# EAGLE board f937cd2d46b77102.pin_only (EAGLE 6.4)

Size 154.94 x 25.4 mm. Coordinates in mm from the lower left corner, seen from the top.
Outline: 0,0 0,25.4 154.94,25.4 154.94,0 0,0
Copper layers (1*16): Top 0.035mm / dielectric 1.5mm / Bottom 0.035mm
Design rules "adafruit_rules_1": minimum track width 8mil, minimum drill 15.5mil, track to track 8mil, track to pad 8mil, pad to pad 8mil, via to via 8mil, smd to smd 8mil, copper to edge 10mil, drill to drill 8mil, minimum pad ring 10mil, minimum via ring 8mil, stop-mask expansion 4mil, vias tented up to drill 25mil, thermal gap 10mil

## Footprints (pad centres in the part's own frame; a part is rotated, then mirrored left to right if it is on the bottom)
0201 = smd 0.3 x 0.3: P$1 -0.3,0; P$2 0.3,0
0402 = smd 0.5 x 0.6: 1 -0.5,0; 2 0.5,0
0603 = smd 0.6 x 0.9: 1 -0.75,0; 2 0.75,0
0805 = smd 1.2 x 1.3: 1 -1.05,0; 2 1.05,0
1206 = smd 0.9 x 1.6: 1 -1.45,0; 2 1.45,0
1210 = smd 1 x 2.8: 1 -1.5,0; 2 1.5,0
2010 = smd 1 x 2.8: P$1 -2.3,0; P$2 2.3,0
DPAK = smd 1.6 x 3: 1 -2.28,-5.31; 3 2.28,-5.31 | smd 4.826 x 5.715: 4 0,1.588
D2PAK = smd 1.6 x 3.5: 1 -2.54,-8.275; 3 2.54,-8.275 | smd 12.2 x 9.75: TAB 0,2
SOT223 = smd 1.219 x 2.235: 1 -2.311,-3.099; 2 0,-3.099; 3 2.311,-3.099 | smd 3.6 x 2.2: 4 0,3.099
SOT89 = smd 0.58 x 1.2: 1 -1.5,-1.8; 2 0,-1.8; 3 1.5,-1.8 | smd 2 x 2: 4 0,1.3
SOT23-5 = smd 0.55 x 1.2: 1 -0.95,-1.3; 2 0,-1.3; 3 0.95,-1.3; 4 0.95,1.3; 5 -0.95,1.3
SOT23-3 = smd 0.8 x 0.9: 1 -0.95,-1; 2 0.95,-1; 3 0,1.1
SC70 = smd 0.4 x 0.75: 1 -0.65,-0.825; 2 0,-0.825; 3 0.65,-0.825; 4 0.65,0.825; 5 -0.65,0.825
CRYSTAL-SMD-5X3.2 = smd 1.8 x 1.2: 1 -2,-1.2; 2 2,-1.2; 3 2,1.2; 4 -2,1.2
CRYSTAL-SMD-3.2X2.5 = smd 1.4 x 1.2: 1 -1.2,-0.95; 2 1.2,-0.95; 3 1.2,0.95; 4 -1.2,0.95
CRYSTAL-SMD-2.5X2 = smd 1.05 x 0.9: 1 -0.795,-0.6; 2 0.795,-0.6; 3 0.795,0.6; 4 -0.795,0.6
HC49UP = smd 5.334 x 1.93: 1 -4.826,0; 2 4.826,0
XTAL-2X1.2 = smd 1 x 1.4: P$1 -0.85,0; P$2 0.85,0
MICROMELF-R = smd 0.8 x 1.2: A 0.8,0; C -0.8,0
SC79_INFINEON = smd 0.35 x 0.35: A 0.675,0; C -0.675,0
SMA-DIODE = smd 1.27 x 1.47: A -2.15,0; C 2.15,0
SMB-DIODE = smd 2.4 x 2.4: A 2.2,0; C -2.2,0
SMC = smd 2.8 x 3.8: A 3.7,0; C -3.7,0
ALL-HOLES = hole 3.26: 43.004,-1.63 | hole 2.91: 39.118,-1.455 | hole 2.59: 35.569,-1.295 | hole 2.3: 32.324,-1.15 | hole 2.05: 29.349,-1.025 | hole 1.83: 26.608,-0.915 | hole 1.63: 24.078,-0.815 | hole 1.45: 21.738,-0.725 | hole 1.29: 19.569,-0.645 | hole 1.15: 17.549,-0.575 | hole 1.02: 15.664,-0.51 | hole 0.912: 13.898,-0.456 | hole 0.812: 12.236,-0.406 | hole 0.723: 10.668,-0.361 | hole 0.644: 9.144,-0.322 | hole 0.573: 7.62,-0.286 | hole 0.511: 6.096,-0.256 | hole 0.455: 4.572,-0.228 | hole 0.405: 3.048,-0.203 | hole 0.361: 1.524,-0.18 | hole 0.321: 0,-0.161
SOD-128 = smd 1.4 x 2.1: A 2.2,0; C -2.2,0
SOD-323 = smd 0.63 x 0.83: 1 -1.15,0; 2 1.15,0
SOD80C = smd 1.4 x 1.8: A 1.7,0; C -1.7,0
QFN-24 = smd 0.8 x 0.25: 1 -2,1.25; 2 -2,0.75; 3 -2,0.25; 4 -2,-0.25; 5 -2,-0.75; 6 -2,-1.25; 13 2,-1.25; 14 2,-0.75; 15 2,-0.25; 16 2,0.25; 17 2,0.75; 18 2,1.25 | smd 0.25 x 0.8: 7 -1.25,-2; 8 -0.75,-2; 9 -0.25,-2; 10 0.25,-2; 11 0.75,-2; 12 1.25,-2; 19 1.25,2; 20 0.75,2; 21 0.25,2; 22 -0.25,2; 23 -0.75,2; 24 -1.25,2
TSSOP16 = smd 0.35 x 1.6: 1 -2.225,-2.85; 2 -1.575,-2.85; 3 -0.925,-2.85; 4 -0.275,-2.85; 5 0.375,-2.85; 6 1.025,-2.85; 7 1.675,-2.85; 8 2.325,-2.85; 9 2.325,3.05; 10 1.675,3.05; 11 1.025,3.05; 12 0.375,3.05; 13 -0.275,3.05; 14 -0.925,3.05; 15 -1.575,3.05; 16 -2.225,3.05
SO08 = smd 0.61 x 2.21: 1 -1.905,-2.616; 2 -0.635,-2.616; 3 0.635,-2.616; 4 1.905,-2.616; 5 1.905,2.616; 6 0.635,2.616; 7 -0.635,2.616; 8 -1.905,2.616
TQFP32-5MM = smd 1.143 x 0.254: 1 -3.5,1.75; 2 -3.5,1.25; 3 -3.5,0.75; 4 -3.5,0.25; 5 -3.5,-0.25; 6 -3.5,-0.75; 7 -3.5,-1.25; 8 -3.5,-1.75; 17 3.5,-1.75; 18 3.5,-1.25; 19 3.5,-0.75; 20 3.5,-0.25; 21 3.5,0.25; 22 3.5,0.75; 23 3.5,1.25; 24 3.5,1.75 | smd 0.254 x 1.143: 9 -1.75,-3.5; 10 -1.25,-3.5; 11 -0.75,-3.5; 12 -0.25,-3.5; 13 0.25,-3.5; 14 0.75,-3.5; 15 1.25,-3.5; 16 1.75,-3.5; 25 1.75,3.5; 26 1.25,3.5; 27 0.75,3.5; 28 0.25,3.5; 29 -0.25,3.5; 30 -0.75,3.5; 31 -1.25,3.5; 32 -1.75,3.5
TQFP100 = smd 1.5 x 0.3: 1 -8,6; 2 -8,5.5; 3 -8,5; 4 -8,4.5; 5 -8,4; 6 -8,3.5; 7 -8,3; 8 -8,2.5; 9 -8,2; 10 -8,1.5; 11 -8,1; 12 -8,0.5; 13 -8,0; 14 -8,-0.5; 15 -8,-1; 16 -8,-1.5; 17 -8,-2; 18 -8,-2.5; 19 -8,-3; 20 -8,-3.5; 21 -8,-4; 22 -8,-4.5; 23 -8,-5; 24 -8,-5.5; 25 -8,-6; 51 8,-6; 52 8,-5.5; 53 8,-5; 54 8,-4.5; 55 8,-4; 56 8,-3.5; 57 8,-3; 58 8,-2.5; 59 8,-2; 60 8,-1.5; 61 8,-1; 62 8,-0.5; 63 8,0; 64 8,0.5; 65 8,1; 66 8,1.5; 67 8,2; 68 8,2.5; 69 8,3; 70 8,3.5; 71 8,4; 72 8,4.5; 73 8,5; 74 8,5.5; 75 8,6 | smd 0.3 x 1.5: 26 -6,-8; 27 -5.5,-8; 28 -5,-8; 29 -4.5,-8; 30 -4,-8; 31 -3.5,-8; 32 -3,-8; 33 -2.5,-8; 34 -2,-8; 35 -1.5,-8; 36 -1,-8; 37 -0.5,-8; 38 0,-8; 39 0.5,-8; 40 1,-8; 41 1.5,-8; 42 2,-8; 43 2.5,-8; 44 3,-8; 45 3.5,-8; 46 4,-8; 47 4.5,-8; 48 5,-8; 49 5.5,-8; 50 6,-8; 76 6,8; 77 5.5,8; 78 5,8; 79 4.5,8; 80 4,8; 81 3.5,8; 82 3,8; 83 2.5,8; 84 2,8; 85 1.5,8; 86 1,8; 87 0.5,8; 88 0,8; 89 -0.5,8; 90 -1,8; 91 -1.5,8; 92 -2,8; 93 -2.5,8; 94 -3,8; 95 -3.5,8; 96 -4,8; 97 -4.5,8; 98 -5,8; 99 -5.5,8; 100 -6,8
TSOP-66 = smd 0.35 x 0.8: P$1 -10.4,-5.7; P$2 -9.75,-5.7; P$3 -9.1,-5.7; P$4 -8.45,-5.7; P$5 -7.8,-5.7; P$6 -7.15,-5.7; P$7 -6.5,-5.7; P$8 -5.85,-5.7; P$9 -5.2,-5.7; P$10 -4.55,-5.7; P$11 -3.9,-5.7; P$12 -3.25,-5.7; P$13 -2.6,-5.7; P$14 -1.95,-5.7; P$15 -1.3,-5.7; P$16 -0.65,-5.7; P$17 0,-5.7; P$18 0.65,-5.7; P$19 1.3,-5.7; P$20 1.95,-5.7; P$21 2.6,-5.7; P$22 3.25,-5.7; P$23 3.9,-5.7; P$24 4.55,-5.7; P$25 5.2,-5.7; P$26 5.85,-5.7; P$27 6.5,-5.7; P$28 7.15,-5.7; P$29 7.8,-5.7; P$30 8.45,-5.7; P$31 9.1,-5.7; P$32 9.75,-5.7; P$33 10.4,-5.7; P$34 10.4,5.7; P$35 9.75,5.7; P$36 9.1,5.7; P$37 8.45,5.7; P$38 7.8,5.7; P$39 7.15,5.7; P$40 6.5,5.7; P$41 5.85,5.7; P$42 5.2,5.7; P$43 4.55,5.7; P$44 3.9,5.7; P$45 3.25,5.7; P$46 2.6,5.7; P$47 1.95,5.7; P$48 1.3,5.7; P$49 0.65,5.7; P$50 0,5.7; P$51 -0.65,5.7; P$52 -1.3,5.7; P$53 -1.95,5.7; P$54 -2.6,5.7; P$55 -3.25,5.7; P$56 -3.9,5.7; P$57 -4.55,5.7; P$58 -5.2,5.7; P$59 -5.85,5.7; P$60 -6.5,5.7; P$61 -7.15,5.7; P$62 -7.8,5.7; P$63 -8.45,5.7; P$64 -9.1,5.7; P$65 -9.75,5.7; P$66 -10.4,5.7
BGA-0.8MM-P-19X19 = smd 0.35 x 0.35: P$1 -4.4,-4.4; P$2 -4.4,-3.6; P$3 -3.6,-3.6; P$4 -3.6,-4.4; P$5 -2.8,-4.4; P$6 -2.8,-3.6; P$7 -4.4,-2.8; P$8 -3.6,-2.8; P$9 -2.8,-2.8; P$10 -4.4,-2; P$11 -3.6,-2; P$12 -2.8,-2; P$13 -2,-2; P$14 -2,-2.8; P$15 -2,-3.6; P$16 -2,-4.4; P$17 -4.4,-1.2; P$18 -3.6,-1.2; P$19 -2.8,-1.2; P$20 -2,-1.2; P$21 -1.2,-1.2; P$22 -1.2,-2; P$23 -1.2,-2.8; P$24 -1.2,-3.6; P$25 -1.2,-4.4; P$26 -3.6,-7.6; P$27 -2.8,-7.6; P$28 -3.6,-6.8; P$29 -2.8,-6.8; P$30 -3.6,-6; P$31 -2.8,-6; P$32 -2,-6; P$33 -2,-6.8; P$34 -2,-7.6; P$35 -3.6,-5.2; P$36 -2.8,-5.2; P$37 -2,-5.2; P$38 -1.2,-5.2; P$39 -1.2,-6; P$40 -1.2,-6.8; P$41 -1.2,-7.6; P$42 -7.6,-3.6; P$43 -6.8,-3.6; P$44 -7.6,-2.8; P$45 -6.8,-2.8; P$46 -7.6,-2; P$47 -6.8,-2; P$48 -6,-2; P$49 -6,-2.8; P$50 -6,-3.6; P$51 -7.6,-1.2; P$52 -6.8,-1.2; P$53 -6,-1.2; P$54 -5.2,-1.2; P$55 -5.2,-2; P$56 -5.2,-2.8; P$57 -5.2,-3.6; P$58 -7.6,-7.6; P$59 -6.8,-7.6; P$60 -7.6,-6.8; P$61 -6.8,-6.8; P$62 -7.6,-6; P$63 -6.8,-6; P$64 -6,-6; P$65 -6,-6.8; P$66 -6,-7.6; P$67 -7.6,-5.2; P$68 -6.8,-5.2; P$69 -6,-5.2; P$70 -5.2,-5.2; P$71 -5.2,-6; P$72 -5.2,-6.8; P$73 -5.2,-7.6; P$74 -7.6,-4.4; P$75 -6.8,-4.4; P$76 -6,-4.4; P$77 -5.2,-4.4; P$78 -4.4,-5.2; P$79 -4.4,-6; P$80 -4.4,-6.8; P$81 -4.4,-7.6; P$82 2.8,-4.4; P$83 2.8,-3.6; P$84 3.6,-3.6; P$85 3.6,-4.4; P$86 4.4,-4.4; P$87 4.4,-3.6; P$88 2.8,-2.8; P$89 3.6,-2.8; P$90 4.4,-2.8; P$91 2.8,-2; P$92 3.6,-2; P$93 4.4,-2; P$94 5.2,-2; P$95 5.2,-2.8; P$96 5.2,-3.6; P$97 5.2,-4.4; P$98 2.8,-1.2; P$99 3.6,-1.2; P$100 4.4,-1.2; P$101 5.2,-1.2; P$102 6,-1.2; P$103 6,-2; P$104 6,-2.8; P$105 6,-3.6; P$106 6,-4.4; P$107 3.6,-7.6; P$108 4.4,-7.6; P$109 3.6,-6.8; P$110 4.4,-6.8; P$111 3.6,-6; P$112 4.4,-6; P$113 5.2,-6; P$114 5.2,-6.8; P$115 5.2,-7.6; P$116 3.6,-5.2; P$117 4.4,-5.2; P$118 5.2,-5.2; P$119 6,-5.2; P$120 6,-6; P$121 6,-6.8; P$122 6,-7.6; P$123 -0.4,-3.6; P$124 0.4,-3.6; P$125 -0.4,-2.8; P$126 0.4,-2.8; P$127 -0.4,-2; P$128 0.4,-2; P$129 1.2,-2; P$130 1.2,-2.8; P$131 1.2,-3.6; P$132 -0.4,-1.2; P$133 0.4,-1.2; P$134 1.2,-1.2; P$135 2,-1.2; P$136 2,-2; P$137 2,-2.8; P$138 2,-3.6; P$139 -0.4,-7.6; P$140 0.4,-7.6; P$141 -0.4,-6.8; P$142 0.4,-6.8; P$143 -0.4,-6; P$144 0.4,-6; P$145 1.2,-6; P$146 1.2,-6.8; P$147 1.2,-7.6; P$148 -0.4,-5.2; P$149 0.4,-5.2; P$150 1.2,-5.2; P$151 2,-5.2; P$152 2,-6; P$153 2,-6.8; P$154 2,-7.6; P$155 -0.4,-4.4; P$156 0.4,-4.4; P$157 1.2,-4.4; P$158 2,-4.4; P$159 2.8,-5.2; P$160 2.8,-6; P$161 2.8,-6.8; P$162 2.8,-7.6; P$163 -4.4,2.8; P$164 -4.4,3.6; P$165 -3.6,3.6; P$166 -3.6,2.8; P$167 -2.8,2.8; P$168 -2.8,3.6; P$169 -4.4,4.4; P$170 -3.6,4.4; P$171 -2.8,4.4; P$172 -4.4,5.2; P$173 -3.6,5.2; P$174 -2.8,5.2; P$175 -2,5.2; P$176 -2,4.4; P$177 -2,3.6; P$178 -2,2.8; P$179 -4.4,6; P$180 -3.6,6; P$181 -2.8,6; P$182 -2,6; P$183 -1.2,6; P$184 -1.2,5.2; P$185 -1.2,4.4; P$186 -1.2,3.6; P$187 -1.2,2.8; P$188 -3.6,-0.4; P$189 -2.8,-0.4; P$190 -3.6,0.4; P$191 -2.8,0.4; P$192 -3.6,1.2; P$193 -2.8,1.2; P$194 -2,1.2; P$195 -2,0.4; P$196 -2,-0.4; P$197 -3.6,2; P$198 -2.8,2; P$199 -2,2; P$200 -1.2,2; P$201 -1.2,1.2; P$202 -1.2,0.4; P$203 -1.2,-0.4; P$204 -7.6,3.6; P$205 -6.8,3.6; P$206 -7.6,4.4; P$207 -6.8,4.4; P$208 -7.6,5.2; P$209 -6.8,5.2; P$210 -6,5.2; P$211 -6,4.4; P$212 -6,3.6; P$213 -7.6,6; P$214 -6.8,6; P$215 -6,6; P$216 -5.2,6; P$217 -5.2,5.2; P$218 -5.2,4.4; P$219 -5.2,3.6; P$220 -7.6,-0.4; P$221 -6.8,-0.4; P$222 -7.6,0.4; P$223 -6.8,0.4; P$224 -7.6,1.2; P$225 -6.8,1.2; P$226 -6,1.2; P$227 -6,0.4; P$228 -6,-0.4; P$229 -7.6,2; P$230 -6.8,2; P$231 -6,2; P$232 -5.2,2; P$233 -5.2,1.2; P$234 -5.2,0.4; P$235 -5.2,-0.4; P$236 -7.6,2.8; P$237 -6.8,2.8; P$238 -6,2.8; P$239 -5.2,2.8; P$240 -4.4,2; P$241 -4.4,1.2; P$242 -4.4,0.4; P$243 -4.4,-0.4; P$244 2.8,2.8; P$245 2.8,3.6; P$246 3.6,3.6; P$247 3.6,2.8; P$248 4.4,2.8; P$249 4.4,3.6; P$250 2.8,4.4; P$251 3.6,4.4; P$252 4.4,4.4; P$253 2.8,5.2; P$254 3.6,5.2; P$255 4.4,5.2; P$256 5.2,5.2; P$257 5.2,4.4; P$258 5.2,3.6; P$259 5.2,2.8; P$260 2.8,6; P$261 3.6,6; P$262 4.4,6; P$263 5.2,6; P$264 6,6; P$265 6,5.2; P$266 6,4.4; P$267 6,3.6; P$268 6,2.8; P$269 3.6,-0.4; P$270 4.4,-0.4; P$271 3.6,0.4; P$272 4.4,0.4; P$273 3.6,1.2; P$274 4.4,1.2; P$275 5.2,1.2; P$276 5.2,0.4; P$277 5.2,-0.4; P$278 3.6,2; P$279 4.4,2; P$280 5.2,2; P$281 6,2; P$282 6,1.2; P$283 6,0.4; P$284 6,-0.4; P$285 -0.4,3.6; P$286 0.4,3.6; P$287 -0.4,4.4; P$288 0.4,4.4; P$289 -0.4,5.2; P$290 0.4,5.2; P$291 1.2,5.2; P$292 1.2,4.4; P$293 1.2,3.6; P$294 -0.4,6; P$295 0.4,6; P$296 1.2,6; P$297 2,6; P$298 2,5.2; P$299 2,4.4; P$300 2,3.6; P$301 -0.4,-0.4; P$302 0.4,-0.4; P$303 -0.4,0.4; P$304 0.4,0.4; P$305 -0.4,1.2; P$306 0.4,1.2; P$307 1.2,1.2; P$308 1.2,0.4; P$309 1.2,-0.4; P$310 -0.4,2; P$311 0.4,2; P$312 1.2,2; P$313 2,2; P$314 2,1.2; P$315 2,0.4; P$316 2,-0.4; P$317 -0.4,2.8; P$318 0.4,2.8; P$319 1.2,2.8; P$320 2,2.8; P$321 2.8,2; P$322 2.8,1.2; P$323 2.8,0.4; P$324 2.8,-0.4; P$325 -4.4,6.8; P$326 -3.6,6.8; P$327 -2.8,6.8; P$328 -4.4,7.6; P$329 -3.6,7.6; P$330 -2.8,7.6; P$331 -2,7.6; P$332 -2,6.8; P$338 -1.2,7.6; P$339 -1.2,6.8; P$340 -7.6,6.8; P$341 -6.8,6.8; P$342 -7.6,7.6; P$343 -6.8,7.6; P$344 -6,7.6; P$345 -6,6.8; P$350 -5.2,7.6; P$351 -5.2,6.8; P$352 2.8,6.8; P$353 3.6,6.8; P$354 4.4,6.8; P$355 2.8,7.6; P$356 3.6,7.6; P$357 4.4,7.6; P$358 5.2,7.6; P$359 5.2,6.8; P$365 6,7.6; P$366 6,6.8; P$367 -0.4,6.8; P$368 0.4,6.8; P$369 -0.4,7.6; P$370 0.4,7.6; P$371 1.2,7.6; P$372 1.2,6.8; P$377 2,7.6; P$378 2,6.8; P$379 6.8,-4.4; P$380 6.8,-3.6; P$381 6.8,-2.8; P$382 6.8,-2; P$383 7.6,-2; P$384 7.6,-2.8; P$385 7.6,-3.6; P$386 7.6,-4.4; P$387 6.8,-1.2; P$388 7.6,-1.2; P$394 6.8,-7.6; P$395 6.8,-6.8; P$396 6.8,-6; P$397 7.6,-6; P$398 7.6,-6.8; P$399 7.6,-7.6; P$400 6.8,-5.2; P$401 7.6,-5.2; P$406 6.8,2.8; P$407 6.8,3.6; P$408 6.8,4.4; P$409 6.8,5.2; P$410 7.6,5.2; P$411 7.6,4.4; P$412 7.6,3.6; P$413 7.6,2.8; P$414 6.8,6; P$415 7.6,6; P$421 6.8,-0.4; P$422 6.8,0.4; P$423 6.8,1.2; P$424 7.6,1.2; P$425 7.6,0.4; P$426 7.6,-0.4; P$427 6.8,2; P$428 7.6,2; P$433 6.8,6.8; P$434 6.8,7.6; P$435 7.6,7.6; P$436 7.6,6.8
TQFP-100-12X12MM = smd 1.5 x 0.2: 1 -6.7,4.8; 2 -6.7,4.4; 3 -6.7,4; 4 -6.7,3.6; 5 -6.7,3.2; 6 -6.7,2.8; 7 -6.7,2.4; 8 -6.7,2; 9 -6.7,1.6; 10 -6.7,1.2; 11 -6.7,0.8; 12 -6.7,0.4; 13 -6.7,0; 14 -6.7,-0.4; 15 -6.7,-0.8; 16 -6.7,-1.2; 17 -6.7,-1.6; 18 -6.7,-2; 19 -6.7,-2.4; 20 -6.7,-2.8; 21 -6.7,-3.2; 22 -6.7,-3.6; 23 -6.7,-4; 24 -6.7,-4.4; 25 -6.7,-4.8; 51 6.7,-4.8; 52 6.7,-4.4; 53 6.7,-4; 54 6.7,-3.6; 55 6.7,-3.2; 56 6.7,-2.8; 57 6.7,-2.4; 58 6.7,-2; 59 6.7,-1.6; 60 6.7,-1.2; 61 6.7,-0.8; 62 6.7,-0.4; 63 6.7,0; 64 6.7,0.4; 65 6.7,0.8; 66 6.7,1.2; 67 6.7,1.6; 68 6.7,2; 69 6.7,2.4; 70 6.7,2.8; 71 6.7,3.2; 72 6.7,3.6; 73 6.7,4; 74 6.7,4.4; 75 6.7,4.8 | smd 0.2 x 1.5: 26 -4.8,-6.7; 27 -4.4,-6.7; 28 -4,-6.7; 29 -3.6,-6.7; 30 -3.2,-6.7; 31 -2.8,-6.7; 32 -2.4,-6.7; 33 -2,-6.7; 34 -1.6,-6.7; 35 -1.2,-6.7; 36 -0.8,-6.7; 37 -0.4,-6.7; 38 0,-6.7; 39 0.4,-6.7; 40 0.8,-6.7; 41 1.2,-6.7; 42 1.6,-6.7; 43 2,-6.7; 44 2.4,-6.7; 45 2.8,-6.7; 46 3.2,-6.7; 47 3.6,-6.7; 48 4,-6.7; 49 4.4,-6.7; 50 4.8,-6.7; 76 4.8,6.7; 77 4.4,6.7; 78 4,6.7; 79 3.6,6.7; 80 3.2,6.7; 81 2.8,6.7; 82 2.4,6.7; 83 2,6.7; 84 1.6,6.7; 85 1.2,6.7; 86 0.8,6.7; 87 0.4,6.7; 88 0,6.7; 89 -0.4,6.7; 90 -0.8,6.7; 91 -1.2,6.7; 92 -1.6,6.7; 93 -2,6.7; 94 -2.4,6.7; 95 -2.8,6.7; 96 -3.2,6.7; 97 -3.6,6.7; 98 -4,6.7; 99 -4.4,6.7; 100 -4.8,6.7
TQFP32-08 = smd 1.27 x 0.559: 1 -4.293,2.8; 2 -4.293,2; 3 -4.293,1.2; 4 -4.293,0.4; 5 -4.293,-0.4; 6 -4.293,-1.2; 7 -4.293,-2; 8 -4.293,-2.8; 17 4.293,-2.8; 18 4.293,-2; 19 4.293,-1.2; 20 4.293,-0.4; 21 4.293,0.4; 22 4.293,1.2; 23 4.293,2; 24 4.293,2.8 | smd 0.559 x 1.27: 9 -2.8,-4.293; 10 -2,-4.293; 11 -1.2,-4.293; 12 -0.4,-4.293; 13 0.4,-4.293; 14 1.2,-4.293; 15 2,-4.293; 16 2.8,-4.293; 25 2.8,4.293; 26 2,4.293; 27 1.2,4.293; 28 0.4,4.293; 29 -0.4,4.293; 30 -1.2,4.293; 31 -2,4.293; 32 -2.8,4.293
BGA-96-14X8MM = smd 0.45 x 0.45: P$1 1.6,6; P$2 2.4,6; P$3 3.2,6; P$4 1.6,5.2; P$5 2.4,5.2; P$6 3.2,5.2; P$7 1.6,4.4; P$8 2.4,4.4; P$9 3.2,4.4; P$10 1.6,3.6; P$11 2.4,3.6; P$12 3.2,3.6; P$13 1.6,2.8; P$14 2.4,2.8; P$15 3.2,2.8; P$16 1.6,2; P$17 2.4,2; P$18 3.2,2; P$19 1.6,1.2; P$20 2.4,1.2; P$21 3.2,1.2; P$22 1.6,0.4; P$23 2.4,0.4; P$24 3.2,0.4; P$25 1.6,-0.4; P$26 2.4,-0.4; P$27 3.2,-0.4; P$28 1.6,-1.2; P$29 2.4,-1.2; P$30 3.2,-1.2; P$31 1.6,-2; P$32 2.4,-2; P$33 3.2,-2; P$34 1.6,-2.8; P$35 2.4,-2.8; P$36 3.2,-2.8; P$37 1.6,-3.6; P$38 2.4,-3.6; P$39 3.2,-3.6; P$40 1.6,-4.4; P$41 2.4,-4.4; P$42 3.2,-4.4; P$43 1.6,-5.2; P$44 2.4,-5.2; P$45 3.2,-5.2; P$46 1.6,-6; P$47 2.4,-6; P$48 3.2,-6; P$49 -3.2,6; P$50 -2.4,6; P$51 -1.6,6; P$52 -3.2,5.2; P$53 -2.4,5.2; P$54 -1.6,5.2; P$55 -3.2,4.4; P$56 -2.4,4.4; P$57 -1.6,4.4; P$58 -3.2,3.6; P$59 -2.4,3.6; P$60 -1.6,3.6; P$61 -3.2,2.8; P$62 -2.4,2.8; P$63 -1.6,2.8; P$64 -3.2,2; P$65 -2.4,2; P$66 -1.6,2; P$67 -3.2,1.2; P$68 -2.4,1.2; P$69 -1.6,1.2; P$70 -3.2,0.4; P$71 -2.4,0.4; P$72 -1.6,0.4; P$73 -3.2,-0.4; P$74 -2.4,-0.4; P$75 -1.6,-0.4; P$76 -3.2,-1.2; P$77 -2.4,-1.2; P$78 -1.6,-1.2; P$79 -3.2,-2; P$80 -2.4,-2; P$81 -1.6,-2; P$82 -3.2,-2.8; P$83 -2.4,-2.8; P$84 -1.6,-2.8; P$85 -3.2,-3.6; P$86 -2.4,-3.6; P$87 -1.6,-3.6; P$88 -3.2,-4.4; P$89 -2.4,-4.4; P$90 -1.6,-4.4; P$91 -3.2,-5.2; P$92 -2.4,-5.2; P$93 -1.6,-5.2; P$94 -3.2,-6; P$95 -2.4,-6; P$96 -1.6,-6

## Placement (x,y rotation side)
E$1  [EDGE-MILLIMETERS]  1.2,0 0 top
E$2  [EDGE-MILLIMETERS]  11.2,0 0 top
E$3  [EDGE-MILLIMETERS]  21.2,0 0 top
E$4  [EDGE-MILLIMETERS]  31.2,0 0 top
E$5  [EDGE-MILLIMETERS]  41.2,0 0 top
E$6  [EDGE-MILLIMETERS]  51.2,0 0 top
E$7  [EDGE-MILLIMETERS]  61.2,0 0 top
E$8  [EDGE-MILLIMETERS]  71.2,0 0 top
E$9  [EDGE-MILLIMETERS]  81.2,0 0 top
E$10  [EDGE-MILLIMETERS]  91.2,0 0 top
E$11  [EDGE-MILLIMETERS]  101.2,0 0 top
E$12  [EDGE-MILLIMETERS]  111.2,0 0 top
E$13  [EDGE-MILLIMETERS]  121.2,0 0 top
E$14  [EDGE-MILLIMETERS]  131.2,0 0 top
E$15  [EDGE-MILLIMETERS]  141.2,0 0 top
E$16  [0201]  19.05,10.46 90 top
E$17  [EDGE-INCHES-EIGTH]  1.27,25.4 0 top
E$18  [EDGE-INCHES-EIGTH]  26.67,25.4 0 top
E$19  [EDGE-INCHES-EIGTH]  52.07,25.4 0 top
E$20  [EDGE-INCHES-EIGTH]  77.47,25.4 0 top
E$21  [EDGE-INCHES-EIGTH]  102.87,25.4 0 top
E$22  [EDGE-INCHES-EIGTH]  128.27,25.4 0 top
E$23  [0402]  20.57,10.16 90 top
E$24  [0603]  22.1,9.86 90 top
E$25  [0805]  23.62,9.27 90 top
E$26  [1206]  25.58,9.02 90 top
E$27  [1210]  28.3,8.92 270 top
E$28  [2010]  31.62,8.13 90 top
E$29  [DPAK]  74.93,14.1 0 top
E$30  [D2PAK]  85.09,14.22 0 top
E$31  [SOT223]  67.56,9.65 0 top
E$32  [SOT89]  67.56,18.03 0 top
E$33  [SOT23-5]  61.98,13.46 0 top
E$34  [SOT23-3]  61.98,18.8 0 top
E$35  [SC70]  61.98,8.13 0 top
E$36  [CRYSTAL-SMD-5X3.2]  94.51,16.89 90 top
E$37  [CRYSTAL-SMD-3.2X2.5]  100.84,17.88 90 top
E$38  [CRYSTAL-SMD-2.5X2]  106.58,18.49 90 top
E$39  [HC49UP]  100.33,7.87 0 top
E$40  [XTAL-2X1.2]  106.43,12.7 0 top
E$41  [MICROMELF-R]  36.07,6.55 90 top
E$42  [SC79_INFINEON]  34.54,6.2 90 top
E$43  [SMA-DIODE]  45.87,8.15 270 top
E$44  [SMB-DIODE]  49.78,8.76 90 top
E$45  [SMC]  55.35,10.44 90 top
E$46  [ALL-HOLES]  109.22,19.3 0 top
E$47  [SOD-128]  42.67,8.28 90 top
E$48  [SOD-323]  37.85,6.81 270 top
E$49  [SOD80C]  39.88,7.75 90 top
E$50  [NMOS-SYMB]  144.78,8.13 0 top
E$51  [PMOS-SYMB]  136.91,8.13 0 top
E$52  [DIODE-SYMB]  147.07,14.22 0 top
E$53  [LED-GUIDE]  135.89,13.97 270 top
E$54  [NPN-SYMB]  129.29,6.86 0 top
E$55  [QFN-24]  112.78,14.73 0 top
E$56  [TSSOP16]  112.78,7.87 270 top
E$57  [SO08]  121.16,6.86 270 top
E$58  [TQFP32-5MM]  121.16,13.97 0 top
E$59  [PNP-SYMB]  129.29,14.22 0 top
E$60  [0201]  19.05,5.79 90 top
E$61  [0402]  20.57,6.1 90 top
E$62  [0603]  22.1,6.38 90 top
E$63  [0201]  19.05,8.13 90 top
E$65  [TQFP100]  55.63,12.7 0 bottom
E$66  [TSOP-66]  7.62,12.7 90 bottom
E$67  [BGA-0.8MM-P-19X19]  35.81,12.7 0 bottom
E$68  [TQFP-100-12X12MM]  74.42,12.7 0 bottom
E$69  [TQFP32-08]  89.41,12.7 0 bottom
E$70  [TQFP32-5MM]  101.09,12.7 0 bottom
E$71  [BGA-96-14X8MM]  20.57,12.7 0 bottom
E$72  [ADAFRUIT-LOGO-0.5IN]  153.42,2.03 0 bottom

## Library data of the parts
E$1-E$63 E$65-E$72 = Reference Ruler

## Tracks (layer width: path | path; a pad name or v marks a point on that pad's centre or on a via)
(copper drawn outside any net)
  shapes: Top area x8

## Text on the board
Bottom: BGA 20X20 | one PCB to RULER them all | BGA | QFP x32 / 0.8mm Pitch | QFP x100 / 0.4mm Pitch | DDR3 RAM | QFP x100 / 0.5mm Pitch | QFP x32 / 0.5mm Pitch | 0.8mm Pitch | TSOP-66 / 0.65mm Pitch | 0.65mm / Pitch
tPlace: 1/8 | 6 | 3 | 0 | 1 | 2 | SOT89 | XTAL/OSC | 4 | 5 | AWG | 28 | 27 | 26 | 25 | 24 | 23 | 22 | 21 | 20 | 19 | 18 | 17 | 16 | 15 | 14 | 13 | 12 | 11 | 10 | 9 | 8 | Trace Width (mil) | 6 | Common Diodes / and Transistors | 8 | SOT23 | 2.5X2 | 3.2X2.4 | 10 | 12 | SMB | 2X1.2 | QFN | QFP | SOD128 | SMC | 5X3.2 | 18 | 0201(0603) / 0402(1005) / 0603(1608) / 0805(2012) | 1206(3216) | 1210(3225) | 2010(5025) | SOD80 | MiniMELF | SMA | DPAK | 24 | D2PAK | 80 | SOD323 | SOT223 | 30 | SC79 | MicroMELF | 60 | 40 | SMD R/C/L | Imperial (Metric) | HC49 | SC70 | SSOP | 50 | SOIC | Font Size | 40mil | 0 | 1 | 2 | 3 | 4 | 5 | 6 | 7 | 9 | 10 | 11 | 12 | 13 | 14 | 15 | 8
bStop: BGA 20X20 | one PCB to RULER them all | BGA | QFP x32 / 0.8mm Pitch | QFP x100 / 0.4mm Pitch | DDR3 RAM | QFP x100 / 0.5mm Pitch | QFP x32 / 0.5mm Pitch | 0.8mm Pitch | TSOP-66 / 0.65mm Pitch | 0.65mm / Pitch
